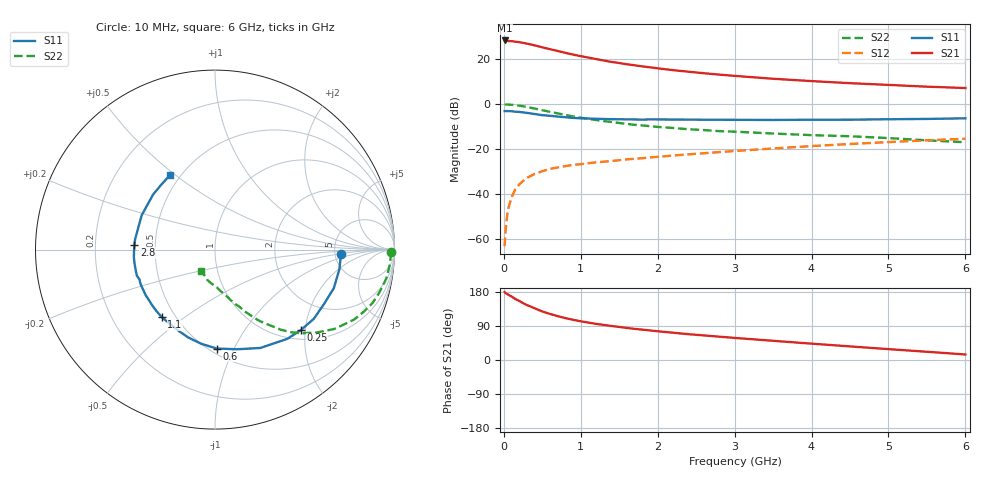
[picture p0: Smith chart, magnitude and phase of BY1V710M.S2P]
! SIEMENS Small Signal Semiconductors
! BFY420
! Si NPN RF SIEGET Grounded Emitter Transistor in MICRO-X
! VCE = 1.75 V  IC = 10 mA
! Common Emitter S-Parameters:  October  1996
# GHz  S  MA  R  50
!  f  S11  S21  S12  S22
! GHz  MAG  ANG  MAG  ANG  MAG  ANG  MAG  ANG
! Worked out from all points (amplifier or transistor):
!   36 points, 10 MHz to 6 GHz, reference 50 ohm
!   highest |S21| = 28.3 dB at 10 MHz (marker M1)
!   |S21| within 3 dB of that: start of sweep to 492.8 MHz
!   unconditionally stable (mu >= 1): 2.492 GHz to end of sweep
!   at 250 MHz: K = 0.19, MSG = 30.7 dB, |S12| = -34.1 dB
!   at 1.4 GHz: K = 0.76, MSG = 22.0 dB, |S12| = -25.3 dB
!   at 6 GHz: K = 1.11, MAG = 9.3 dB, |S12| = -15.4 dB
!   S11 on the Smith chart (normalised r, x): 10 MHz: 5.63, -0.54; 250 MHz: 1.20, -1.89; 600 MHz: 0.54, -0.86; 1.1 GHz: 0.42, -0.41; 2.8 GHz: 0.38, +0.02; 6 GHz: 0.44, +0.47
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0.01  0.7008 -2.0  25.98 179.2  0.0007 91.6  0.9793 -0.8
0.02  0.7011 -4.1  25.95 176.7  0.0014 85.8  0.9801 -1.7
0.05  0.7017 -9.0  25.33 173.1  0.0043 82.7  0.9784 -4.7
0.1  0.6959 -18.0  25.05 167.7  0.0085 82.4  0.9674 -9.7
0.15  0.679 -26.5  24.4 160.8  0.0129 75.6  0.948 -14.3
0.2  0.6721 -35.0  23.84 155.9  0.0165 75.1  0.927 -18.7
0.25  0.6556 -43.3  22.97 150.1  0.0197 69.4  0.8961 -22.9
0.3  0.6398 -51.0  22.09 145.0  0.023 67.4  0.8667 -26.8
0.4  0.6036 -65.2  20.27 136.5  0.0281 61.9  0.7988 -33.6
0.5  0.5689 -77.4  18.26 128.0  0.0324 57.9  0.7331 -39.0
0.6  0.5513 -89.0  16.64 121.6  0.0365 55.3  0.6749 -43.7
0.8  0.5112 -107.2  13.79 110.6  0.0419 50.4  0.5754 -50.7
0.9  0.4959 -114.2  12.6 106.0  0.0447 49.1  0.5346 -53.1
1.1  0.4795 -128.2  10.81 98.6  0.0489 48.4  0.4704 -57.9
1.3  0.4681 -138.1  9.317 92.5  0.0528 47.5  0.4202 -61.2
1.6  0.458 -151.3  7.688 84.5  0.0593 46.8  0.3636 -65.6
2.2  0.455 -169.7  5.691 72.0  0.0722 45.9  0.2958 -72.6
2.8  0.4495 176.7  4.534 61.6  0.086 44.4  0.2513 -78.4
3.5  0.4449 163.4  3.664 50.7  0.1036 41.2  0.2225 -84.6
4.5  0.4518 146.4  2.923 35.9  0.1302 34.9  0.1935 -94.4
5.5  0.4696 129.5  2.443 21.7  0.1573 26.9  0.1568 -111.3
6  0.4842 121.5  2.281 14.6  0.1701 22.5  0.1426 -123.1
